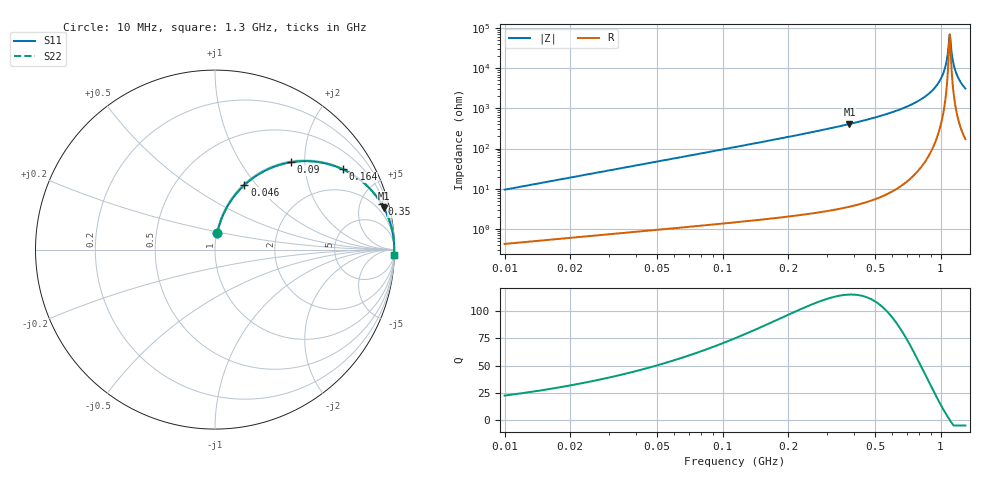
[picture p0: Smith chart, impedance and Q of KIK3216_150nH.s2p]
!version-2
!date-01.2022
!Series
# MHz S RI R 50
!Freq ReS11 ImS11 ReS21 ImS21 ReS12 ImS12 ReS22 ImS22
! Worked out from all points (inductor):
!   646 points, 10 MHz to 1.3 GHz, reference 50 ohm
!   read as one part in series: L = 150 nH near 16 MHz
!   highest Q = 115 at 382 MHz (marker M1), where L = 170 nH
!   self-resonance near 1.102 GHz
!   S11 on the Smith chart (normalised r, x): 10 MHz: 1.01, +0.19; 46 MHz: 1.02, +0.87; 90 MHz: 1.03, +1.71; 164 MHz: 1.04, +3.16; 350 MHz: 1.06, +7.34; 1.3 GHz: 4, -62
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10  0.0129 0.0927  0.9871 -0.0927  0.9871 -0.0927  0.0129 0.0927
26  0.0623 0.2284  0.9377 -0.2284  0.9377 -0.2284  0.0623 0.2284
46  0.1638 0.3599  0.8362 -0.3599  0.8362 -0.3599  0.1638 0.3599
90  0.4229 0.4866  0.5771 -0.4866  0.5771 -0.4866  0.4229 0.4866
164  0.712 0.4472  0.288 -0.4472  0.288 -0.4472  0.712 0.4472
226  0.8293 0.3713  0.1707 -0.3713  0.1707 -0.3713  0.8293 0.3713
350  0.9289 0.2526  0.0711 -0.2526  0.0711 -0.2526  0.9289 0.2526
382  0.9419 0.2297  0.0581 -0.2297  0.0581 -0.2297  0.9419 0.2297
440  0.959 0.194  0.041 -0.194  0.041 -0.194  0.959 0.194
656  0.988 0.1031  0.012 -0.1031  0.012 -0.1031  0.988 0.1031
870  0.9967 0.0458  0.00332 -0.0458  0.00332 -0.0458  0.9967 0.0458
956  0.998 0.0274  0.00203 -0.0274  0.00203 -0.0274  0.998 0.0274
1018  0.9984 0.0153  0.00157 -0.0153  0.00157 -0.0153  0.9984 0.0153
1060  0.9986 0.0075  0.00144 -0.0075  0.00144 -0.0075  0.9986 0.0075
1074  0.9986 0.00498  0.00142 -0.00498  0.00142 -0.00498  0.9986 0.00498
1086  0.9986 0.00285  0.00142 -0.00285  0.00142 -0.00285  0.9986 0.00285
1098  0.9986 0.000741  0.00143 -0.000741  0.00143 -0.000741  0.9986 0.000741
1104  0.9986 -0.000305  0.00144 0.000305  0.00144 0.000305  0.9986 -0.000305
1132  0.9985 -0.00511  0.0015 0.00511  0.0015 0.00511  0.9985 -0.00511
1166  0.9984 -0.0108  0.00164 0.0108  0.00164 0.0108  0.9984 -0.0108
1222  0.998 -0.0198  0.002 0.0198  0.002 0.0198  0.998 -0.0198
1300  0.9972 -0.0318  0.00276 0.0318  0.00276 0.0318  0.9972 -0.0318
